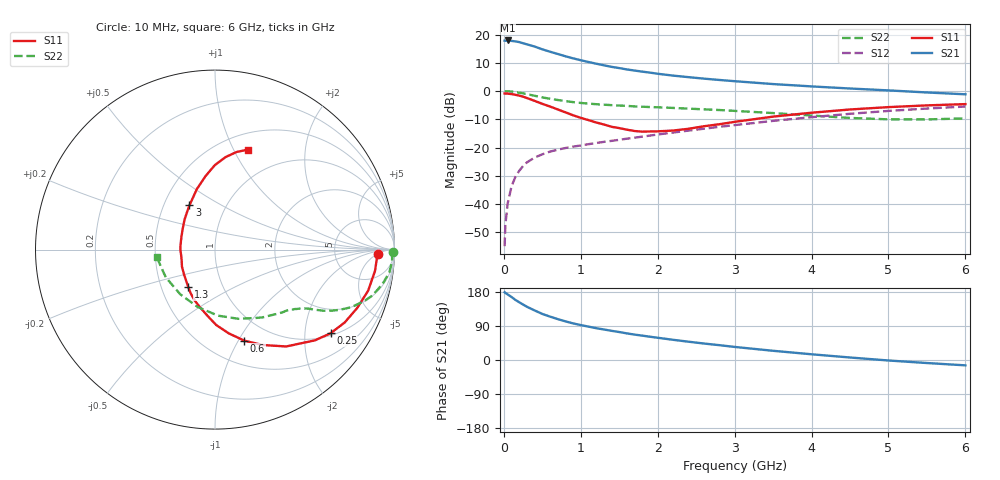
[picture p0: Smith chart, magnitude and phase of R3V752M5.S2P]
! SIEMENS Small Signal Semiconductors
! BFR181
! Si NPN RF Bipolar Junction Transistor in SOT23
! VCE = 0.75 V  IC = 2.5 mA
! Common Emitter S-Parameters:  May  1996
# GHz  S  MA  R  50
!  f  S11  S21  S12  S22
! GHz  MAG  ANG  MAG  ANG  MAG  ANG  MAG  ANG
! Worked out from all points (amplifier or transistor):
!   36 points, 10 MHz to 6 GHz, reference 50 ohm
!   highest |S21| = 17.9 dB at 50 MHz (marker M1)
!   |S21| within 3 dB of that: start of sweep to 486.2 MHz
!   unconditionally stable (mu >= 1): 1.319 GHz to 3.61 GHz
!   at 250 MHz: K = 0.28, MSG = 21.7 dB, |S12| = -26.5 dB
!   at 1.4 GHz: K = 1.03, MAG = 12.0 dB, |S12| = -17.6 dB
!   at 6 GHz: K = 0.91, MSG = 2.2 dB, |S12| = -5.5 dB
!   S11 on the Smith chart (normalised r, x): 10 MHz: 19, -5; 250 MHz: 1.07, -2.71; 600 MHz: 0.75, -1.06; 1.3 GHz: 0.68, -0.31; 3 GHz: 0.67, +0.36; 6 GHz: 0.67, +1.14
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0.01  0.9071 -1.6  7.781 178.8  0.0018 90.2  0.9936 -0.8
0.02  0.9034 -2.9  7.746 177.0  0.0043 85.0  0.9872 -1.5
0.05  0.8994 -7.6  7.846 173.0  0.0103 87.4  0.9887 -3.7
0.1  0.8835 -15.0  7.702 166.3  0.0206 81.8  0.9796 -7.3
0.15  0.8565 -22.3  7.543 158.6  0.0303 76.8  0.9588 -10.7
0.2  0.8291 -29.3  7.348 152.4  0.0388 73.3  0.9338 -13.8
0.25  0.795 -35.9  6.997 146.3  0.0471 69.9  0.9093 -16.6
0.3  0.7525 -42.2  6.694 140.5  0.0546 67.4  0.8815 -18.9
0.4  0.6697 -53.7  6.125 130.8  0.0666 62.2  0.8246 -22.9
0.5  0.5933 -63.6  5.468 121.6  0.0759 58.5  0.7715 -25.8
0.6  0.5326 -72.2  4.962 114.5  0.0848 55.8  0.7302 -27.8
0.8  0.4202 -89.1  4.121 102.0  0.0981 53.1  0.6634 -30.5
0.9  0.3726 -96.2  3.785 96.6  0.1038 52.9  0.6367 -31.5
1.1  0.3058 -111.7  3.264 88.1  0.1147 52.6  0.5994 -33.2
1.3  0.2563 -125.6  2.852 80.6  0.1261 52.4  0.5733 -35.0
1.7  0.1961 -161.1  2.302 67.0  0.1494 53.5  0.5344 -38.6
2.2  0.1999 159.5  1.874 53.3  0.1843 53.7  0.5023 -45.1
3  0.2847 120.0  1.493 34.5  0.2493 51.3  0.4454 -58.7
3.5  0.3526 106.6  1.328 24.3  0.2963 48.1  0.4075 -71.2
4.5  0.4716 90.0  1.108 6.6  0.3953 38.3  0.3343 -106.5
5.5  0.5572 77.5  0.943 -8.0  0.49 25.8  0.3147 -150.7
6  0.5871 71.7  0.875 -14.1  0.5316 18.7  0.3276 -172.6
